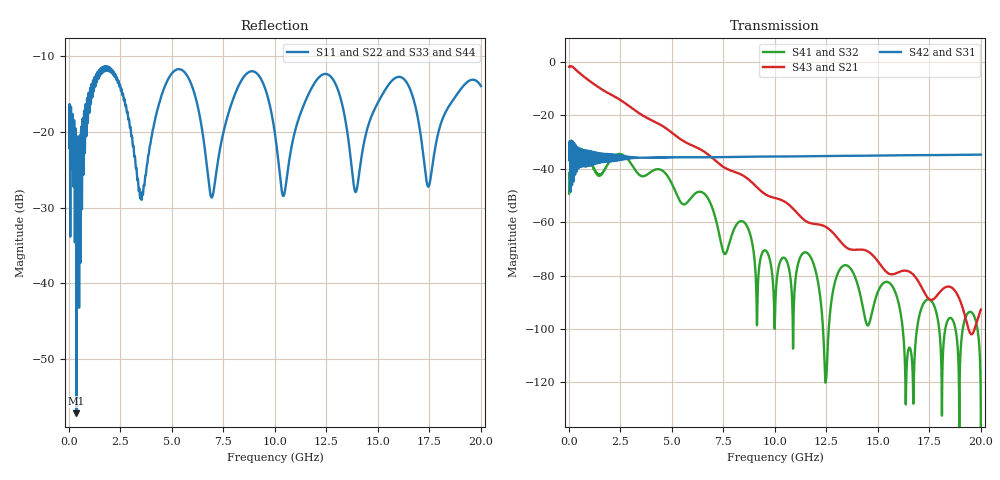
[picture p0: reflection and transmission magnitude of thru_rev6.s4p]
! Created Wed Aug 18 17:01:24 2004
# hz S ma R 50
! 4 Port Network Data from SP1.SP block
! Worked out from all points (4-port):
!   3999 points, 10 MHz to 20 GHz, reference 50 ohm
!   strongest paths, dB at 10 MHz, 5.005 GHz, 10.01 GHz, 15.01 GHz, 20 GHz:
!     S42: -36.8, -35.7, -35.4, -35.0, -34.7
!     S31: -36.8, -35.7, -35.4, -35.0, -34.7
!     S43: -1.7, -26.5, -50.9, -74.7, -92.7
!     S21: -1.7, -26.5, -50.9, -74.7, -92.7
!     S41: -49.2, -45.7, -95.3, -86.0, -142.8
!     S32: -49.2, -45.7, -95.3, -86.0, -142.8
!   lowest |S11| = -57.2 dB at 360 MHz (marker M1), VSWR 1.00, Z = 49.9 - j0.0229 ohm
!   |S11| at or under -10 dB: start of sweep to end of sweep
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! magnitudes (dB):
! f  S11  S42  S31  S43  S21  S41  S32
! 10 MHz  -22.1  -36.8  -36.8  -1.7  -1.7  -49.2  -49.2
! 360 MHz  -57.2  -35.1  -35.1  -3.1  -3.1  -33.9  -33.9
! 1.755 GHz  -11.3  -37.3  -37.3  -11.0  -11.0  -39.9  -39.9
! 6.52 GHz  -20.7  -35.7  -35.7  -33.3  -33.3  -49.0  -49.0
! 9.135 GHz  -12.3  -35.4  -35.4  -46.9  -46.9  -96.7  -96.7
! 10.41 GHz  -28.5  -35.4  -35.4  -52.0  -52.0  -73.3  -73.3
! 20 GHz  -13.9  -34.7  -34.7  -92.7  -92.7  -142.8  -142.8
